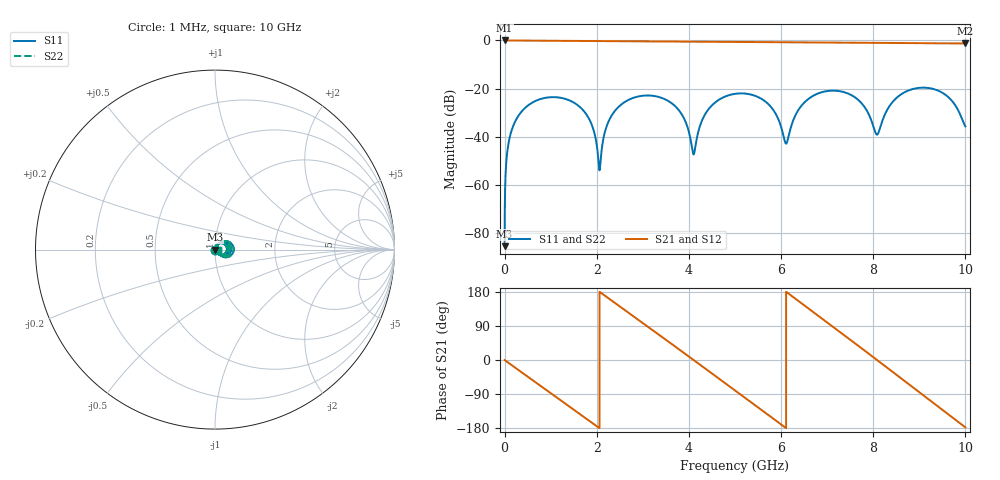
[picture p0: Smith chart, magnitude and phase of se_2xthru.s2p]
!Created with skrf (http://scikit-rf.org).
# GHz S RI R 50.0
!freq ReS11 ImS11 ReS21 ImS21 ReS12 ImS12 ReS22 ImS22
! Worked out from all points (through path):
!   10000 points, 1 MHz to 10 GHz, reference 50 ohm
!   highest |S21| = 0.00 dB at 1 MHz (marker M1); lowest = -1.2 dB at 10 GHz (marker M2)
!   group delay of S21, straight-line fit = 249 ps
!   lowest |S11| = -85.6 dB at 1 MHz (marker M3), VSWR 1.00, Z = 50 + j0.00517 ohm
!   |S11| at or under -10 dB: start of sweep to end of sweep
!   |S22| runs from -85.6 to -19.6 dB; largest |S21 - S12| = 5.5e-16
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0.001  -9.58e-06 5.17e-05  0.9999 -0.00158  0.9999 -0.00158  -9.58e-06 5.17e-05
0.096  0.000133 0.00818  0.9874 -0.1472  0.9874 -0.1472  0.000133 0.00818
0.355  0.0131 0.0291  0.8507 -0.5147  0.8507 -0.5147  0.0131 0.0291
1.011  0.0654 0.00989  0.0284 -0.9831  0.0284 -0.9831  0.0654 0.00989
1.668  0.0263 -0.0281  -0.8051 -0.5515  -0.8051 -0.5515  0.0263 -0.0281
1.901  0.00754 -0.0149  -0.9445 -0.2358  -0.9445 -0.2358  0.00754 -0.0149
2.062  0.00196 0.000345  -0.9717 0.00171  -0.9717 0.00171  0.00196 0.000345
2.216  0.00408 0.016  -0.9423 0.2284  -0.9423 0.2284  0.00408 0.016
2.441  0.0192 0.0335  -0.8067 0.5318  -0.8067 0.5318  0.0192 0.0335
3.334  0.065 -0.017  0.3556 0.8838  0.3556 0.8838  0.065 -0.017
3.825  0.0188 -0.0248  0.8614 0.3955  0.8614 0.3955  0.0188 -0.0248
4.102  0.00423 0.000413  0.9449 0.000285  0.9449 0.000285  0.00423 0.000413
4.414  0.0172 0.0314  0.8317 -0.4389  0.8317 -0.4389  0.0172 0.0314
5.001  0.0751 0.0195  0.1576 -0.917  0.1576 -0.917  0.0751 0.0195
5.708  0.0363 -0.033  -0.7428 -0.5471  -0.7428 -0.5471  0.0363 -0.033
6.109  0.00713 0.000503  -0.9186 -0.00141  -0.9186 -0.00141  0.00713 0.000503
6.667  0.0522 0.0435  -0.5768 0.7032  -0.5768 0.7032  0.0522 0.0435
7.537  0.062 -0.0364  0.5744 0.6893  0.5744 0.6893  0.062 -0.0364
8.079  0.011 0.000273  0.8926 0.00531  0.8926 0.00531  0.011 0.000273
8.334  0.0229 0.0333  0.8166 -0.351  0.8166 -0.351  0.0229 0.0333
9.13  0.104 -0.004  -0.1034 -0.868  -0.1034 -0.868  0.104 -0.004
10  0.0161 -0.00275  -0.8667 -0.0334  -0.8667 -0.0334  0.0161 -0.00275
